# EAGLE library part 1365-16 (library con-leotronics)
DUAL ROW STRAIGHT HEADER 1364 SERIES. 1.27mm x 1.27mm. Without Fixing Post. SMT Source: http://www.leotronics.co.uk/Conexcon/Data%20Sheets/sec.%20A/1364ing.pdf
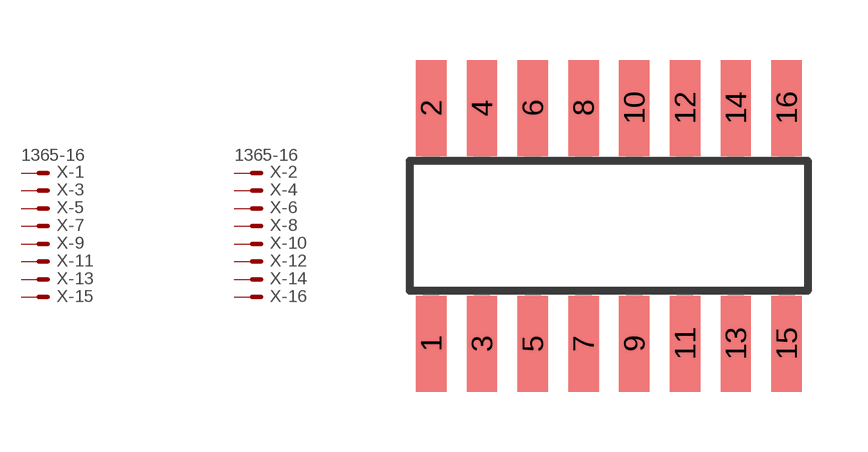
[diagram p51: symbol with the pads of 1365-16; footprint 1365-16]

Designator prefix X; gates -1=MVAL -2=MVAL -3=M -4=M -5=M -6=M -7=M -8=M -9=M -10=M -11=M -12=M -13=M -14=M -15=M -16=M

## 1365-16 (OC_FARNELL: unknown; OC_NEWARK: unknown)  [1365-16]
1  -1:S  pas
2  -2:S  pas
3  -3:S  pas
4  -4:S  pas
5  -5:S  pas
6  -6:S  pas
7  -7:S  pas
8  -8:S  pas
9  -9:S  pas
10  -10:S  pas
11  -11:S  pas
12  -12:S  pas
13  -13:S  pas
14  -14:S  pas
15  -15:S  pas
16  -16:S  pas

## Footprint 1365-16 (pad centres in mm)
DUAL ROW STRAIGHT HEADER 1364 SERIES. 1.27mm x 1.27mm. Without Fixing Post. SMT Source: http://www.leotronics.co.uk/Conexcon/Data%20Sheets/sec.%20A/1364ing.pdf
smd 0.76 x 2.4: 1 -4.445,-2.95; 2 -4.445,2.95; 3 -3.175,-2.95; 4 -3.175,2.95; 5 -1.905,-2.95; 6 -1.905,2.95; 7 -0.635,-2.95; 8 -0.635,2.95; 9 0.635,-2.95; 10 0.635,2.95; 11 1.905,-2.95; 12 1.905,2.95; 13 3.175,-2.95; 14 3.175,2.95; 15 4.445,-2.95; 16 4.445,2.95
